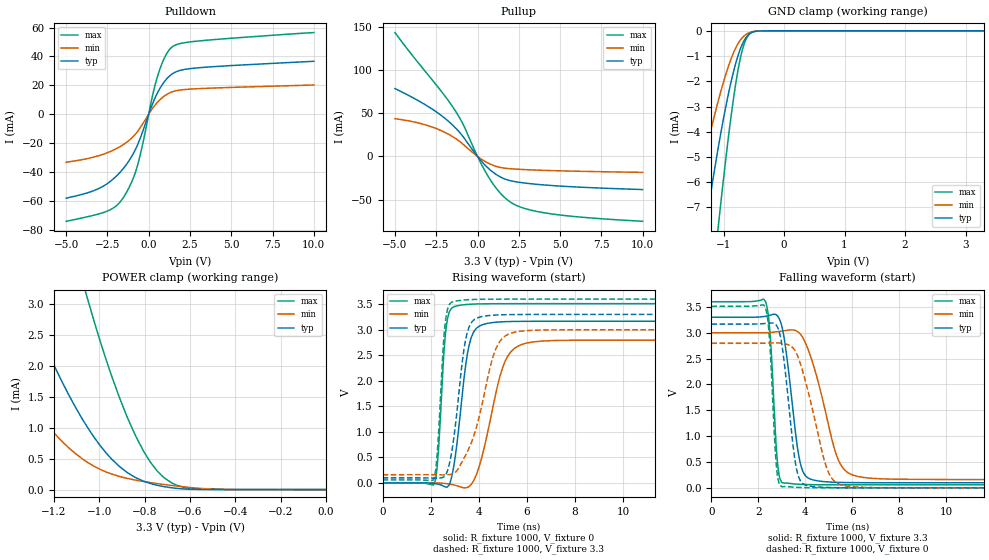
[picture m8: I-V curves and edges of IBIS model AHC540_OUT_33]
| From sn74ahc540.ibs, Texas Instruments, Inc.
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[Model]   AHC540_OUT_33
Model_type  3-state
Enable   Active-Low
Vref =   0
Rref =   1000
Cref =   50p
Vmeas =   1.65
| variable   typ   min   max
C_comp   2.55pF   2.34pF   2.65pF
| C_pullup   3.55pF   2.55pF   4.28pF
| C_pulldown   3.34pF   2.70pF   4.21pF
| C_tri-state   2.55pF   2.34pF   2.65pF
[Temperature Range]   40   100   -40
| Ambient temperature   25   85   -40
[Voltage range]   3.3   3   3.6
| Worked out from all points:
|   slope of the pulldown table from 0 to 0.495 V, typ, clamps not added: 35.5 ohm
|   slope of the pullup table from 0 to 0.495 V, typ, clamps not added: 45.9 ohm
|   GND clamp passes 1 mA (typ) near -0.76 V on its own axis
|   POWER clamp passes 1 mA (typ) near -1.05 V on its own axis
|   rising waveform, R_fixture 1000, V_fixture 0: 20-80 % time 475ps typ, 822ps min, 261ps max; typ from 0 V to 3.17 V
|   falling waveform, R_fixture 1000, V_fixture 3.3: 20-80 % time 505ps typ, 952ps min, 252ps max; typ from 3.3 V to 0.098 V
|   rising waveform, R_fixture 1000, V_fixture 3.3: 20-80 % time 481ps typ, 929ps min, 258ps max; typ from 0.098 V to 3.3 V
|   falling waveform, R_fixture 1000, V_fixture 0: 20-80 % time 456ps typ, 895ps min, 239ps max; typ from 3.17 V to 0 V
[GND Clamp]
| AHC540_OUT_33
|   Voltage   I(typ)   I(min)   I(max)
-5V       -95.67mA   -62.49mA   -121.3mA
-1.555V   -12.25mA   -7.735mA   -19.36mA
-1.3V     -7.837mA   -4.868mA   -12.82mA
-1.275V   -7.436mA   -4.607mA   -12.21mA
-1.08V    -4.531mA   -2.712mA   -7.608mA
-910mV    -2.397mA   -1.344mA   -4.04mA
-785mV    -1.175mA   -614.9uA   -1.899mA
-680mV    -478.4uA   -246.1uA   -680.2uA
-630mV    -269.2uA   -144.6uA   -345.6uA
-555mV    -91.43uA   -56.78uA   -96.81uA
-265mV    -288.9nA   -278nA     -62.51nA
3.3V      9.182nA    24.41nA    44.02nA
[POWER Clamp]
| AHC540_OUT_33
|   Voltage   I(typ)   I(min)   I(max)
-5V       75.68mA    48.36mA    122.9mA
-1.6V     5.955mA    3.194mA    12.64mA
-1.345V   3.264mA    1.609mA    7.645mA
-1.315V   2.988mA    1.452mA    7.116mA
-1.195V   1.98mA     900.5uA    5.136mA
-1.075V   1.146mA    499uA      3.399mA
-1.05V    997.5uA    437uA      3.07mA
-945mV    493.1uA    251.9uA    1.836mA
-840mV    195.2uA    153.7uA    872uA
-715mV    48.2uA     82.85uA    194.4uA
-590mV    4.157uA    30.5uA     16.28uA
-84.45fV  9.182nA    1.38nA     68.2nA
[Pulldown]
| AHC540_OUT_33
|   Voltage   I(typ)   I(min)   I(max)
-5V       -58.22mA   -33.3mA    -74.29mA
-2.425V   -47.47mA   -26.37mA   -66.79mA
-1.89V    -42.15mA   -23.5mA    -62.78mA
-1.435V   -36.16mA   -20.28mA   -55.98mA
-995mV    -28.58mA   -16.15mA   -45.97mA
-665mV    -20.99mA   -11.81mA   -34.99mA
230mV     7.139mA    3.976mA    12.88mA
585mV     15.93mA    8.911mA    28.09mA
1.005V    23.32mA    13.03mA    40.23mA
1.42V     27.88mA    15.47mA    46.64mA
2.975V    32.13mA    17.67mA    50.7mA
10V       36.65mA    20.22mA    56.58mA
[Pullup]
| AHC540_OUT_33
|   Voltage   I(typ)   I(min)   I(max)
-5V       78.49mA    43.61mA    143.3mA
-3.015V   58.01mA    35.68mA    94.8mA
-2.18V    47.14mA    29.65mA    74.97mA
-1.495V   36.02mA    22.72mA    57.08mA
-870mV    22.74mA    13.94mA    37.03mA
10mV      -243.6uA   -145.2uA   -400.6uA
585mV     -12.48mA   -7.165mA   -21.17mA
1.225V    -22.05mA   -12.01mA   -38.99mA
1.86V     -27.43mA   -14.04mA   -51.03mA
2.745V    -30.53mA   -15.13mA   -59.53mA
4.215V    -33.28mA   -16.24mA   -65.75mA
10V       -38.35mA   -18.45mA   -75.06mA
[Ramp]
| AHC540_OUT_33
| variable   typ   min   max
dV/dt_r   1.95/4.92E-10   1.74/8.52E-10   2.13/2.70E-10
dV/dt_f   1.96/5.19E-10   1.74/9.76E-10   2.16/2.61E-10
R_load = 1000
[Rising Waveform]
| AHC540_OUT_33
R_fixture =   1000
C_fixture =   0
L_fixture =   0
V_fixture =   0
V_fixture_min = 0
V_fixture_max = 0
|   Time   V(typ)   V(min)   V(max)
0s        1.497nV    2.529nV    870pV
2.145ns   -11.08mV   712.7uV    -14.44mV
2.295ns   -23.64mV   -517.1uV   467.8mV
2.67ns    -82.03mV   -15.42mV   3.135V
3.27ns    1.53V      -84.2mV    3.483V
3.56ns    2.609V     -81.51mV   3.498V
3.88ns    3.017V     137.6mV    3.505V
5.08ns    3.158V     2.364V     3.511V
6.275ns   3.166V     2.763V     3.511V
50ns      3.167V     2.796V     3.511V
[Falling Waveform]
| AHC540_OUT_33
R_fixture =   1000
C_fixture =   0
L_fixture =   0
V_fixture =   3.3
V_fixture_min = 3
V_fixture_max = 3.6
|   Time   V(typ)   V(min)   V(max)
0s        3.3V       3V         3.6V
2.305ns   3.32V      3.001V     3.6V
2.5ns     3.34V      3.006V     2.959V
2.82ns    3.32V      3.021V     455mV
3.095ns   2.898V     3.039V     91.87mV
3.795ns   456.7mV    2.97V      68.19mV
4.62ns    129.1mV    1.916V     60.62mV
5.49ns    105mV      457.7mV    59.12mV
6.74ns    99.33mV    187.8mV    58.74mV
50ns      98.36mV    160.4mV    58.67mV
[Rising Waveform]
| AHC540_OUT_33
R_fixture =   1000
C_fixture =   0
L_fixture =   0
V_fixture =   3.3
V_fixture_min = 3
V_fixture_max = 3.6
|   Time   V(typ)   V(min)   V(max)
0s        98.36mV    160.4mV    58.67mV
2.11ns    92.8mV     160.3mV    56.06mV
2.265ns   90.95mV    159.4mV    544.6mV
2.62ns    153.8mV    156.8mV    3.188V
3.115ns   1.495V     255.3mV    3.567V
3.405ns   2.677V     501.7mV    3.584V
3.695ns   3.141V     792.5mV    3.592V
4.725ns   3.289V     2.641V     3.599V
5.725ns   3.299V     2.97V      3.6V
50ns      3.3V       3V         3.6V
[Falling Waveform]
| AHC540_OUT_33
R_fixture =   1000
C_fixture =   0
L_fixture =   0
V_fixture =   0
V_fixture_min = 0
V_fixture_max = 0
|   Time   V(typ)   V(min)   V(max)
0s        3.167V     2.796V     3.511V
2.305ns   3.179V     2.8V       3.474V
2.48ns    3.186V     2.802V     2.823V
2.77ns    3.141V     2.805V     398.4mV
3.005ns   2.753V     2.798V     21.19mV
3.625ns   361.6mV    2.598V     10.52mV
4.29ns    28.57mV    1.539V     2.844mV
5.035ns   6.867mV    250.7mV    795.1uV
6.075ns   1.252mV    19.36mV    155.7uV
50ns      -1.512nV   1.134nV    -1.717nV
